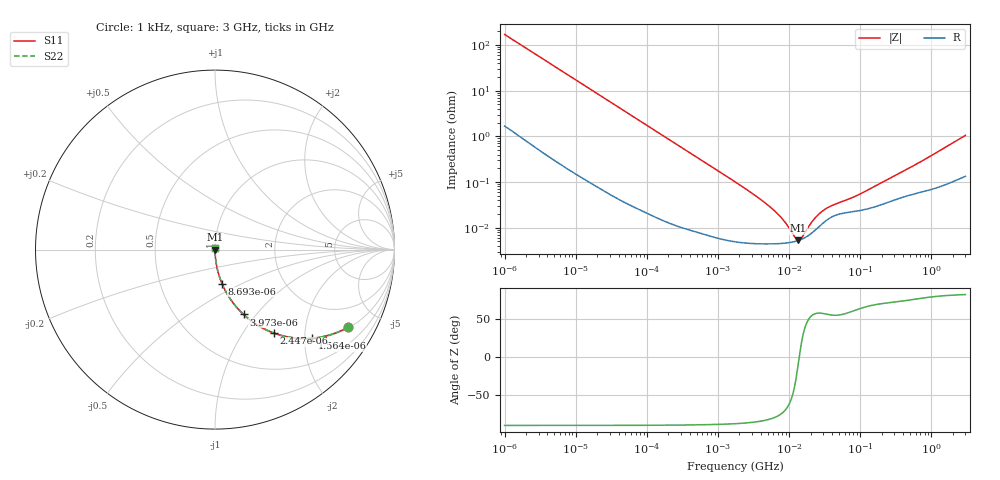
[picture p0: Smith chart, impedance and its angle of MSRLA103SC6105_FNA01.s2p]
! MSRLA103SC6105_FNA01  S-PARAMETER MODEL  ( Standard Model )
! Model Generated by TAIYO YUDEN Corporation (http://www.ty-top.com)
! Version 1.0
! TAIYO YUDEN Control No. 220601
! Copyright(c) 2010 TAIYO YUDEN CO.,LTD. All Rights Reserved.
! Product Description (link to TY-COMPAS)
! https://ds.yuden.co.jp/TYCOMPAS/or/detail?pn=MSRLA103SC6105MFNA01&u=M
! Products Name : Multilayer Ceramic Capacitors
! Characteristics :
!  Capacitance : 1 [uF] , Rated Voltage : 4 [V] , TCC : X6S
!  Case Size : 0.52 x 1.0 / 0.02 x 0.039 [mm/inch] , Thickness : 0.3 / 0.012 [mm/inch]
!  (Conditions: Temperature = 25 [degC] , DC Bias Voltage = 0 [V])
! External Node Assignments :
!  1  o---| |---o  2
! GND o---------o GND
! Frequency Range : 1kHz  -  3GHz  [ 401 STEP ]
# MHZ S RI R 50
! Freq[MHz].  S11 Real  S11 Imag  S21 Real  S21 Imag  S12 Real  S12 Imag  S22 Real  S22 Imag
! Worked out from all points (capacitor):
!   401 points, 1 kHz to 3 GHz, reference 50 ohm
!   read as one part in series: C = 935 nF near 1.077 kHz
!   lowest |Z| = 5.29 mohm at 13.46 MHz (marker M1)
!   series resonance near 13.83 MHz, so ESL is about 140 pH
!   S11 on the Smith chart (normalised r, x): 1 kHz: 1.03, -3.40; 1.564 kHz: 1.02, -2.18; 2.447 kHz: 1.01, -1.40; 3.973 kHz: 1.01, -0.86; 8.693 kHz: 1.00, -0.40; 3 GHz: 1.00, +0.02
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0.001  0.7405 -0.4334  0.2595 0.4334  0.2595 0.4334  0.7405 -0.4334
0.001564  0.5423 -0.4935  0.4577 0.4935  0.4577 0.4935  0.5423 -0.4935
0.002447  0.3292 -0.4654  0.6708 0.4654  0.6708 0.4654  0.3292 -0.4654
0.003973  0.1589 -0.3613  0.8411 0.3613  0.8411 0.3613  0.1589 -0.3613
0.005768  0.0833 -0.272  0.9167 0.272  0.9167 0.272  0.0833 -0.272
0.008693  0.0392 -0.1898  0.9608 0.1898  0.9608 0.1898  0.0392 -0.1898
0.01216  0.0208 -0.1386  0.9792 0.1386  0.9792 0.1386  0.0208 -0.1386
0.033275  0.00319 -0.0519  0.9968 0.0519  0.9968 0.0519  0.00319 -0.0519
0.147855  0.000296 -0.0118  0.9997 0.0118  0.9997 0.0118  0.000296 -0.0118
1.732051  5.01e-05 -0.00101  0.9999 0.00101  0.9999 0.00101  5.01e-05 -0.00101
5.30084  4.42e-05 -0.000288  1 0.000288  1 0.000288  4.42e-05 -0.000288
7.143107  4.48e-05 -0.000184  1 0.000184  1 0.000184  4.48e-05 -0.000184
9.991309  4.71e-05 -8.66e-05  1 8.66e-05  1 8.66e-05  4.71e-05 -8.66e-05
13.46371  5.24e-05 -7.11e-06  0.9999 7.11e-06  0.9999 7.11e-06  5.24e-05 -7.11e-06
17.47891  6.32e-05 6.21e-05  0.9999 -6.21e-05  0.9999 -6.21e-05  6.32e-05 6.21e-05
18.83216  6.81e-05 8.22e-05  0.9999 -8.22e-05  0.9999 -8.22e-05  6.81e-05 8.22e-05
21.06097  7.75e-05 0.000112  0.9999 -0.000112  0.9999 -0.000112  7.75e-05 0.000112
27.34186  0.000111 0.000179  0.9999 -0.000179  0.9999 -0.000179  0.000111 0.000179
35.49586  0.000155 0.000233  0.9998 -0.000233  0.9998 -0.000233  0.000155 0.000233
90.15665  0.000232 0.000453  0.9998 -0.000453  0.9998 -0.000453  0.000232 0.000453
256.0921  0.000369 0.00113  0.9996 -0.00113  0.9996 -0.00113  0.000369 0.00113
3000  0.00144 0.0104  0.9986 -0.0104  0.9986 -0.0104  0.00144 0.0104
